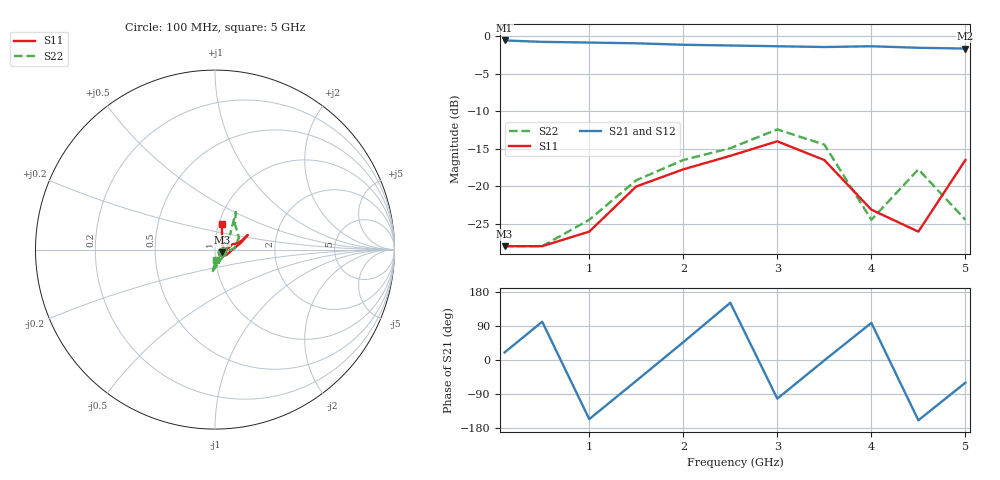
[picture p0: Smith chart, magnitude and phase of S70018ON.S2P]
!  MGS-70018 S PARAMETERS
!  "on" port  LAST UPDATED 07-22-92
# ghz s ma r 50
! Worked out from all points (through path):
!   11 points, 100 MHz to 5 GHz, reference 50 ohm
!   highest |S21| = -0.54 dB at 100 MHz (marker M1); lowest = -1.6 dB at 5 GHz (marker M2)
!   lowest |S11| = -28.0 dB at 100 MHz (marker M3), VSWR 1.08, Z = 53.9 - j1.55 ohm
!   |S11| at or under -10 dB: start of sweep to end of sweep
!   |S22| runs from -28.0 to -12.4 dB; largest |S21 - S12| = 0.031
0.1  0.04 -21.0  0.94 20.0  0.94 20.0  0.04 -22.0
0.5  0.04 -54.0  0.92 101.0  0.92 101.0  0.04 -44.0
1  0.05 -22.0  0.91 -156.0  0.91 -156.0  0.06 -17.0
1.5  0.1 17.0  0.9 -55.0  0.9 -54.0  0.11 5.0
2  0.13 16.0  0.88 47.0  0.88 47.0  0.15 27.0
2.5  0.16 19.0  0.87 151.0  0.86 151.0  0.18 52.0
3  0.2 24.0  0.86 -102.0  0.87 -103.0  0.24 61.0
3.5  0.15 15.0  0.85 -1.0  0.86 1.0  0.19 57.0
4  0.07 -26.0  0.86 98.0  0.87 98.0  0.06 -19.0
4.5  0.05 38.0  0.84 -159.0  0.85 -160.0  0.13 -98.0
5  0.15 75.0  0.83 -60.0  0.85 -61.0  0.06 -83.0
